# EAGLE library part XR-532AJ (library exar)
PULSE DETECTOR
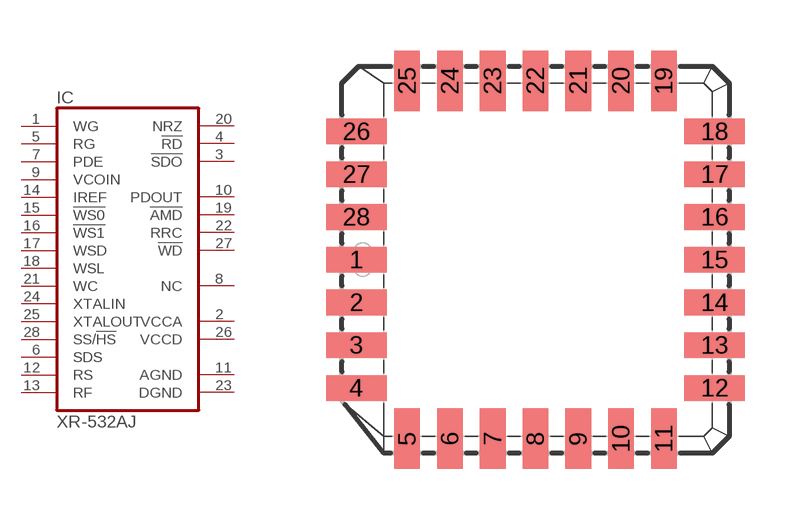
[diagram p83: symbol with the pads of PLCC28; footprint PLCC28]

Designator prefix IC

## XR-532AJ (OC_FARNELL: unknown; OC_NEWARK: unknown)  [PLCC28]
1  WG  in
2  VCCA  pwr
3  !SDO
4  !RD
5  RG  in
6  SDS  in
7  PDE  in
8  NC  nc
9  VCOIN  in
10  PDOUT  out
11  AGND  pwr
12  RS  in
13  RF  in
14  IREF  in
15  !WS0  in
16  !WS1  in
17  WSD  in
18  WSL  in
19  !AMD  out
20  NRZ
21  WC  in
22  RRC  out
23  DGND  pwr
24  XTALIN  in
25  XTALOUT  in
26  VCCD  pwr
27  !WD  out
28  SS/!HS  in

## Footprint PLCC28 (pad centres in mm)
Plastic Leaded Chip Carrier
smd 1.8 x 0.76: 1 -5.32,0; 2 -5.32,-1.27; 3 -5.32,-2.54; 4 -5.32,-3.81; 12 5.32,-3.81; 13 5.32,-2.54; 14 5.32,-1.27; 15 5.32,0; 16 5.32,1.27; 17 5.32,2.54; 18 5.32,3.81; 26 -5.32,3.81; 27 -5.32,2.54; 28 -5.32,1.27
smd 0.76 x 1.8: 5 -3.81,-5.32; 6 -2.54,-5.32; 7 -1.27,-5.32; 8 0,-5.32; 9 1.27,-5.32; 10 2.54,-5.32; 11 3.81,-5.32; 19 3.81,5.32; 20 2.54,5.32; 21 1.27,5.32; 22 0,5.32; 23 -1.27,5.32; 24 -2.54,5.32; 25 -3.81,5.32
